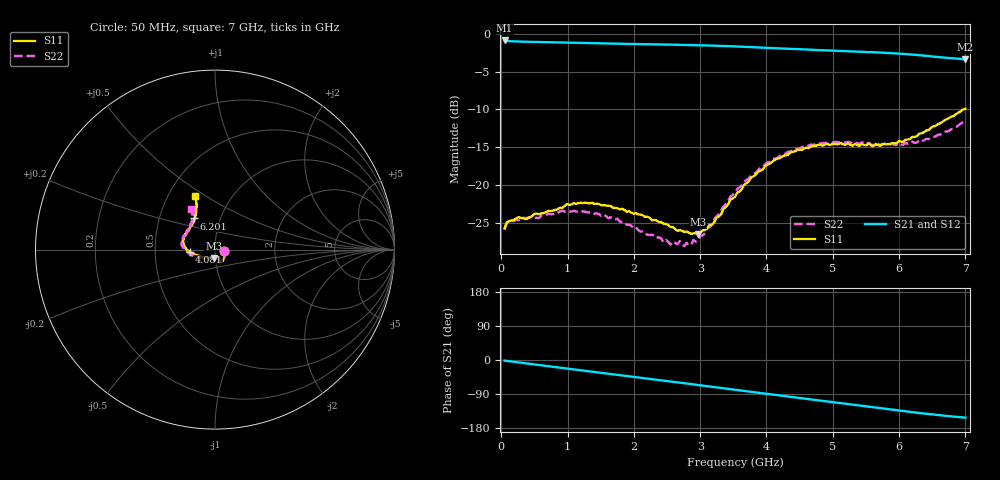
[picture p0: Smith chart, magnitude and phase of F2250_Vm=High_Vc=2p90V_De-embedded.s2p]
! Integrated Device Technology
! Corporate Headquarters
! 6024 Silver Creek Valley Road
! San Jose, CA 95138  USA
! Phone:  1-408-284-8200
! Toll Free:  1-800-223-1366
! Webpage:  http://www.idt.com/
! Timing and RF Division
! 515 Groton Road, Suite 102
! Westford, MA 01886-6024
! Device:  F2250
! Description: Voltage Variable RF Attenuator
! Frequency:  50.0 -  6000.00 MHz
! Package:  3x3 mm Thin QFN Plastic Package: 16 pin
! Ports:  2 RF, 3 DC
!  Pin  1  = GND
!  Pin  2  = NC
!  Pin  3  = RF1  = Port 1
!  Pin  4  = NC
!  Pin  5  = GND
!  Pin  6  = GND
!  Pin  7  = GND
!  Pin  8  = GND
!  Pin  9  = NC
!  Pin 10  = RF2  = Port 2
!  Pin 11  = NC
!  Pin 12  = GND
!  Pin 13  = GND
!  Pin 14  = VCNTRL
!  Pin 15  = VDD
!  Pin 16  = VMODE
! Vcntrl:  2.900 Volts
! Vmode:  +3.300 Volts
! Vdd:  +3.30  Volts
! Current:  1.313 mA
! Data:  The device was measured on a the F2250 evaluation board which has
!  individual transmission lines to the RF pins.  Data was collected
!  using a calibrated network analyzer.  The evaluation board was
!  de-embedded using a TRL calibration technique.
!  The reference plane is the edge of the package pin.
! Misc:  SN 10
!  Action Tracker AT0258
! Date Measured:  2014-11-26
! Date:  2015-10-15  MJV
! Note:
!  Integrated Device Technology supplies this data as a sample of measured
!  data at the package pin for this product.  Your particular data for this
!  product may vary.
!  Data was taken at 25 degrees C.
!  Integrated Device Technology reserves the right to change this data at anytime.
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# GHz S dB R 50
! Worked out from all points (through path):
!   201 points, 50 MHz to 7 GHz, reference 50 ohm
!   highest |S21| = -0.89 dB at 50 MHz (marker M1); lowest = -3.4 dB at 7 GHz (marker M2)
!   group delay of S21, straight-line fit = 61.2 ps
!   lowest |S11| = -26.5 dB at 2.969 GHz (marker M3), VSWR 1.10, Z = 49.1 - j4.62 ohm
!   |S11| at or under -10 dB: start of sweep to 6.967 GHz
!   |S22| runs from -28.0 to -11.5 dB; largest |S21 - S12| = 0.0019
!   S11 on the Smith chart (normalised r, x): 50 MHz: 1.11, -0.02; 4.081 GHz: 0.75, -0.02; 6.201 GHz: 0.75, +0.27; 7 GHz: 0.68, +0.45
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0.05  -25.69 -10.8  -0.89 -1.8  -0.89 -1.8  -25.85 -11.0
0.1195  -24.76 -10.1  -0.99 -3.2  -0.98 -3.2  -24.69 -8.8
0.57125  -23.84 -31.3  -1.10 -13.3  -1.10 -13.3  -24.33 -31.4
0.91875  -23.00 -50.1  -1.17 -21.0  -1.17 -21.1  -23.36 -51.0
1.2315  -22.36 -57.9  -1.24 -27.9  -1.24 -27.9  -23.48 -61.5
1.75275  -23.03 -64.8  -1.33 -39.1  -1.33 -39.1  -24.42 -67.8
2.37825  -24.87 -64.5  -1.42 -52.8  -1.42 -52.8  -26.86 -66.7
2.552  -25.52 -69.5  -1.44 -56.7  -1.44 -56.7  -27.85 -73.1
2.691  -25.92 -77.5  -1.47 -59.8  -1.47 -59.8  -27.37 -80.8
2.7605  -26.17 -79.7  -1.48 -61.3  -1.48 -61.3  -28.05 -85.3
2.969  -26.49 -97.8  -1.52 -66.0  -1.52 -66.0  -27.27 -104.8
3.1775  -25.21 -120.9  -1.57 -70.7  -1.57 -70.7  -25.25 -126.7
3.525  -21.54 -152.8  -1.68 -78.5  -1.68 -78.6  -20.97 -148.7
3.76825  -18.97 -164.8  -1.77 -84.0  -1.77 -84.1  -18.70 -159.6
4.081  -16.95 -175.7  -1.90 -91.0  -1.90 -91.0  -16.72 -171.4
4.4285  -15.54 176.0  -2.03 -98.6  -2.03 -98.6  -15.19 178.7
4.7065  -14.76 169.1  -2.13 -104.8  -2.13 -104.8  -14.68 173.0
5.054  -14.60 160.9  -2.26 -112.5  -2.25 -112.5  -14.27 166.0
5.85325  -14.56 135.0  -2.56 -130.0  -2.56 -130.1  -14.67 147.3
6.20075  -13.62 123.6  -2.77 -137.7  -2.77 -137.8  -14.24 138.2
6.54825  -12.18 115.6  -3.04 -144.7  -3.04 -144.9  -13.58 126.9
7  -9.91 110.7  -3.37 -152.1  -3.37 -152.2  -11.54 120.7
